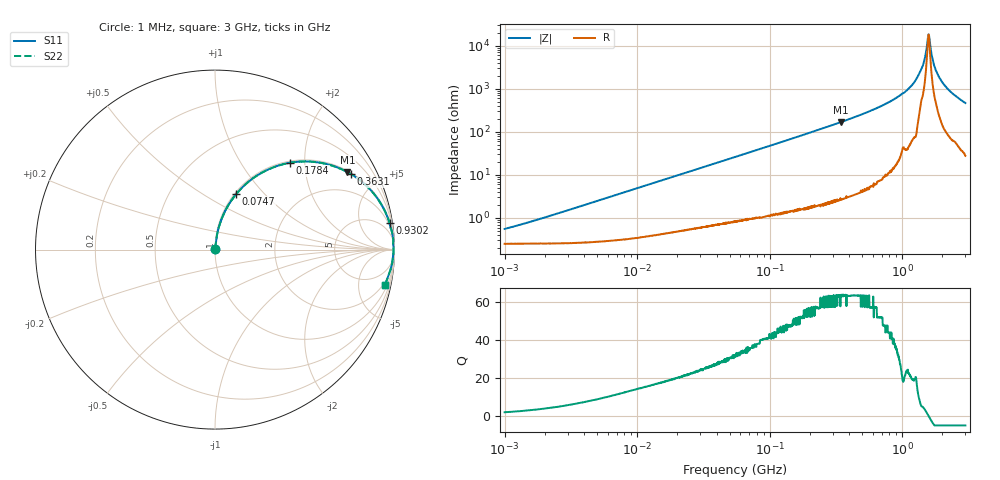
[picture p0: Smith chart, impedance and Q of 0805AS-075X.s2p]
!s-Parameter Generated by FASTRON Sdn. Bhd.
!FASTRON P/N : 0805AS-075X
!Keysight Technologies: E4991B_MY54100416_A.01.15
!Date: Mon Jun 15 12:51:35 2026
!Version  :Rev01  Mon Jun 15 12:51:35 2026
!Data & Calibration Information:
!Freq  S11  S21  S12  S22
!PortZ  Port1:50+j0  Port2:50+j0
!When reading reference impedance value at option line is always used.
! Remarks : This data is being provided solely for informational purposes.
# Hz S dB R 50
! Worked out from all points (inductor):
!   1601 points, 1 MHz to 3 GHz, reference 50 ohm
!   read as one part in series: L = 79 nH near 1.53 MHz
!   highest Q = 63.7 at 345.4 MHz (marker M1), where L = 77.9 nH
!   self-resonance near 1.581 GHz
!   S11 on the Smith chart (normalised r, x): 1 MHz: 1.01, +0.01; 74.7 MHz: 1.02, +0.71; 178.4 MHz: 1.03, +1.69; 363.1 MHz: 1.06, +3.58; 930.2 MHz: 1, +13; 3 GHz: 1.56, -9.34
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1000000  -45.10 62.9  -0.02 -0.3  -0.02 -0.3  -45.10 62.9
3804036  -34.40 80.9  -0.02 -1.1  -0.02 -1.1  -34.40 80.9
1.447069e7  -23.10 82.7  -0.06 -4.0  -0.06 -4.0  -23.10 82.7
5.504702e7  -12.00 73.6  -0.36 -14.6  -0.36 -14.6  -12.00 73.6
7.46963e7  -9.59 69.1  -0.59 -19.3  -0.59 -19.3  -9.59 69.1
1.784169e8  -3.87 49.1  -2.43 -39.8  -2.43 -39.8  -3.87 49.1
2.083556e8  -3.12 44.7  -3.06 -44.3  -3.06 -44.3  -3.12 44.7
3.453811e8  -1.36 30.4  -5.92 -58.7  -5.92 -58.7  -1.36 30.4
3.631036e8  -1.24 29.0  -6.28 -60.1  -6.28 -60.1  -1.24 29.0
7.925923e8  -0.22 11.5  -14.00 -77.2  -14.00 -77.2  -0.22 11.5
9.302341e8  -0.14 8.6  -16.50 -79.6  -16.50 -79.6  -0.14 8.6
1.125055e9  -0.08 5.5  -20.30 -81.9  -20.30 -81.9  -0.08 5.5
1.294266e9  -0.04 3.1  -25.20 -83.2  -25.20 -83.2  -0.04 3.1
1.430499e9  -0.06 1.6  -30.70 -76.6  -30.70 -76.6  -0.06 1.6
1.542004e9  -0.05 0.4  -40.60 -53.7  -40.60 -53.7  -0.05 0.4
1.581072e9  -0.05 0.0  -45.30 -4.5  -45.30 -4.5  -0.05 0.0
1.621129e9  -0.05 -0.4  -41.40 50.6  -41.40 50.6  -0.05 -0.4
1.704314e9  -0.05 -1.2  -33.20 74.0  -33.20 74.0  -0.05 -1.2
1.76507e9  -0.06 -1.8  -29.90 77.2  -29.90 77.2  -0.06 -1.8
1.950859e9  -0.08 -3.5  -24.30 80.1  -24.30 80.1  -0.08 -3.5
2.335937e9  -0.14 -6.7  -18.60 78.6  -18.60 78.6  -0.14 -6.7
3e9  -0.30 -11.9  -13.70 74.7  -13.70 74.7  -0.30 -11.9
